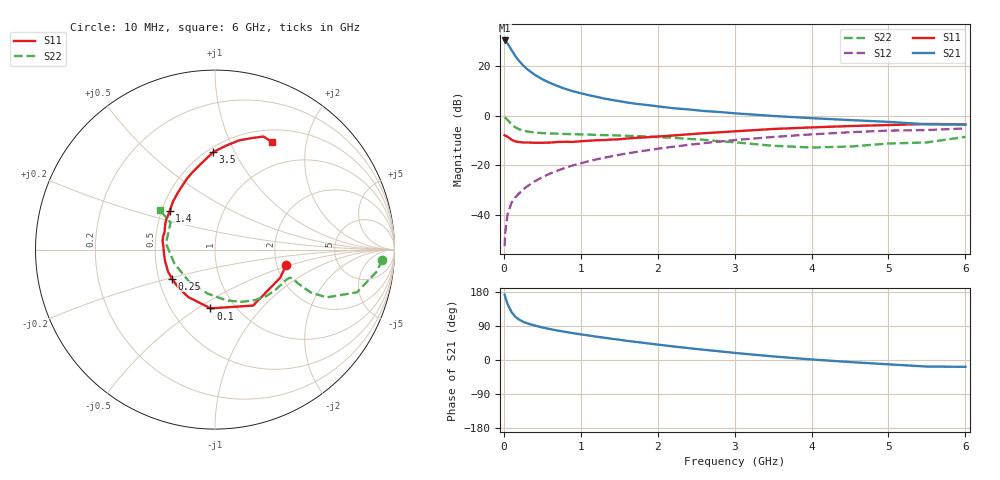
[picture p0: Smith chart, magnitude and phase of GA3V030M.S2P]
! Infineon Technologies  Discrete & RF Semiconductors
! BF775
! Si NPN RF Bipolar Junction Transistor in SOT23
! VCE = 3 V  IC = 30 mA
! Common Emitter S-Parameters:  May  1996
# GHz  S  MA  R  50
!  f  S11  S21  S12  S22
! GHz  MAG  ANG  MAG  ANG  MAG  ANG  MAG  ANG
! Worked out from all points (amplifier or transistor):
!   36 points, 10 MHz to 6 GHz, reference 50 ohm
!   highest |S21| = 30.5 dB at 10 MHz (marker M1)
!   |S21| within 3 dB of that: start of sweep to 83.24 MHz
!   unconditionally stable (mu >= 1): 219.7 MHz to 3.771 GHz; 5.212 GHz to end of sweep
!   at 250 MHz: K = 1.04, MAG = 23.9 dB, |S12| = -29.9 dB
!   at 1.4 GHz: K = 1.19, MAG = 8.8 dB, |S12| = -16.4 dB
!   at 6 GHz: K = 1.01, MAG = 0.0 dB, |S12| = -5.1 dB
!   S11 on the Smith chart (normalised r, x): 10 MHz: 2.24, -0.46; 100 MHz: 0.77, -0.57; 250 MHz: 0.59, -0.21; 1.4 GHz: 0.55, +0.27; 3.5 GHz: 0.54, +0.83; 6 GHz: 0.66, +1.46
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0.01  0.4053 -12.3  33.65 172.6  0.0023 87.2  0.9314 -3.5
0.02  0.3957 -23.4  32.87 165.4  0.0046 76.9  0.9119 -7.5
0.05  0.3772 -55.7  29.06 147.1  0.0105 73.3  0.8266 -16.7
0.1  0.3286 -94.4  21.55 126.7  0.0174 66.7  0.6767 -23.2
0.15  0.3033 -119.6  16.18 114.1  0.0226 65.7  0.5848 -24.1
0.2  0.2944 -134.3  12.87 106.5  0.0271 68.1  0.5346 -23.1
0.25  0.2893 -146.1  10.56 101.1  0.0321 69.0  0.5028 -22.3
0.3  0.2891 -154.5  8.924 97.0  0.0371 70.7  0.4839 -21.5
0.4  0.2854 -166.7  6.818 91.1  0.0472 72.0  0.4614 -20.5
0.5  0.2853 -175.4  5.52 85.8  0.0573 72.9  0.4479 -20.5
0.6  0.2876 177.1  4.648 81.7  0.0678 72.5  0.4403 -21.3
0.7  0.2961 170.6  4.008 77.6  0.0781 72.6  0.4353 -22.2
0.8  0.2983 165.8  3.515 74.2  0.0888 71.8  0.4298 -23.3
0.9  0.2971 160.7  3.148 70.8  0.0996 71.4  0.4256 -24.6
1.1  0.3132 151.8  2.636 64.8  0.1205 70.1  0.4174 -28.1
1.4  0.3314 139.7  2.109 56.1  0.1519 67.5  0.4056 -33.3
1.7  0.3578 130.3  1.771 48.1  0.1837 64.4  0.3911 -39.4
2.2  0.4001 117.0  1.432 35.9  0.2372 58.7  0.3602 -51.3
3.5  0.5429 91.1  0.996 9.5  0.3738 41.3  0.248 -100.0
4.5  0.6227 77.6  0.822 -5.4  0.4665 26.7  0.2391 -160.9
5.5  0.6854 66.8  0.675 -17.3  0.5159 10.7  0.2899 148.8
6  0.678 61.9  0.662 -18.0  0.5579 6.3  0.3759 144.5
